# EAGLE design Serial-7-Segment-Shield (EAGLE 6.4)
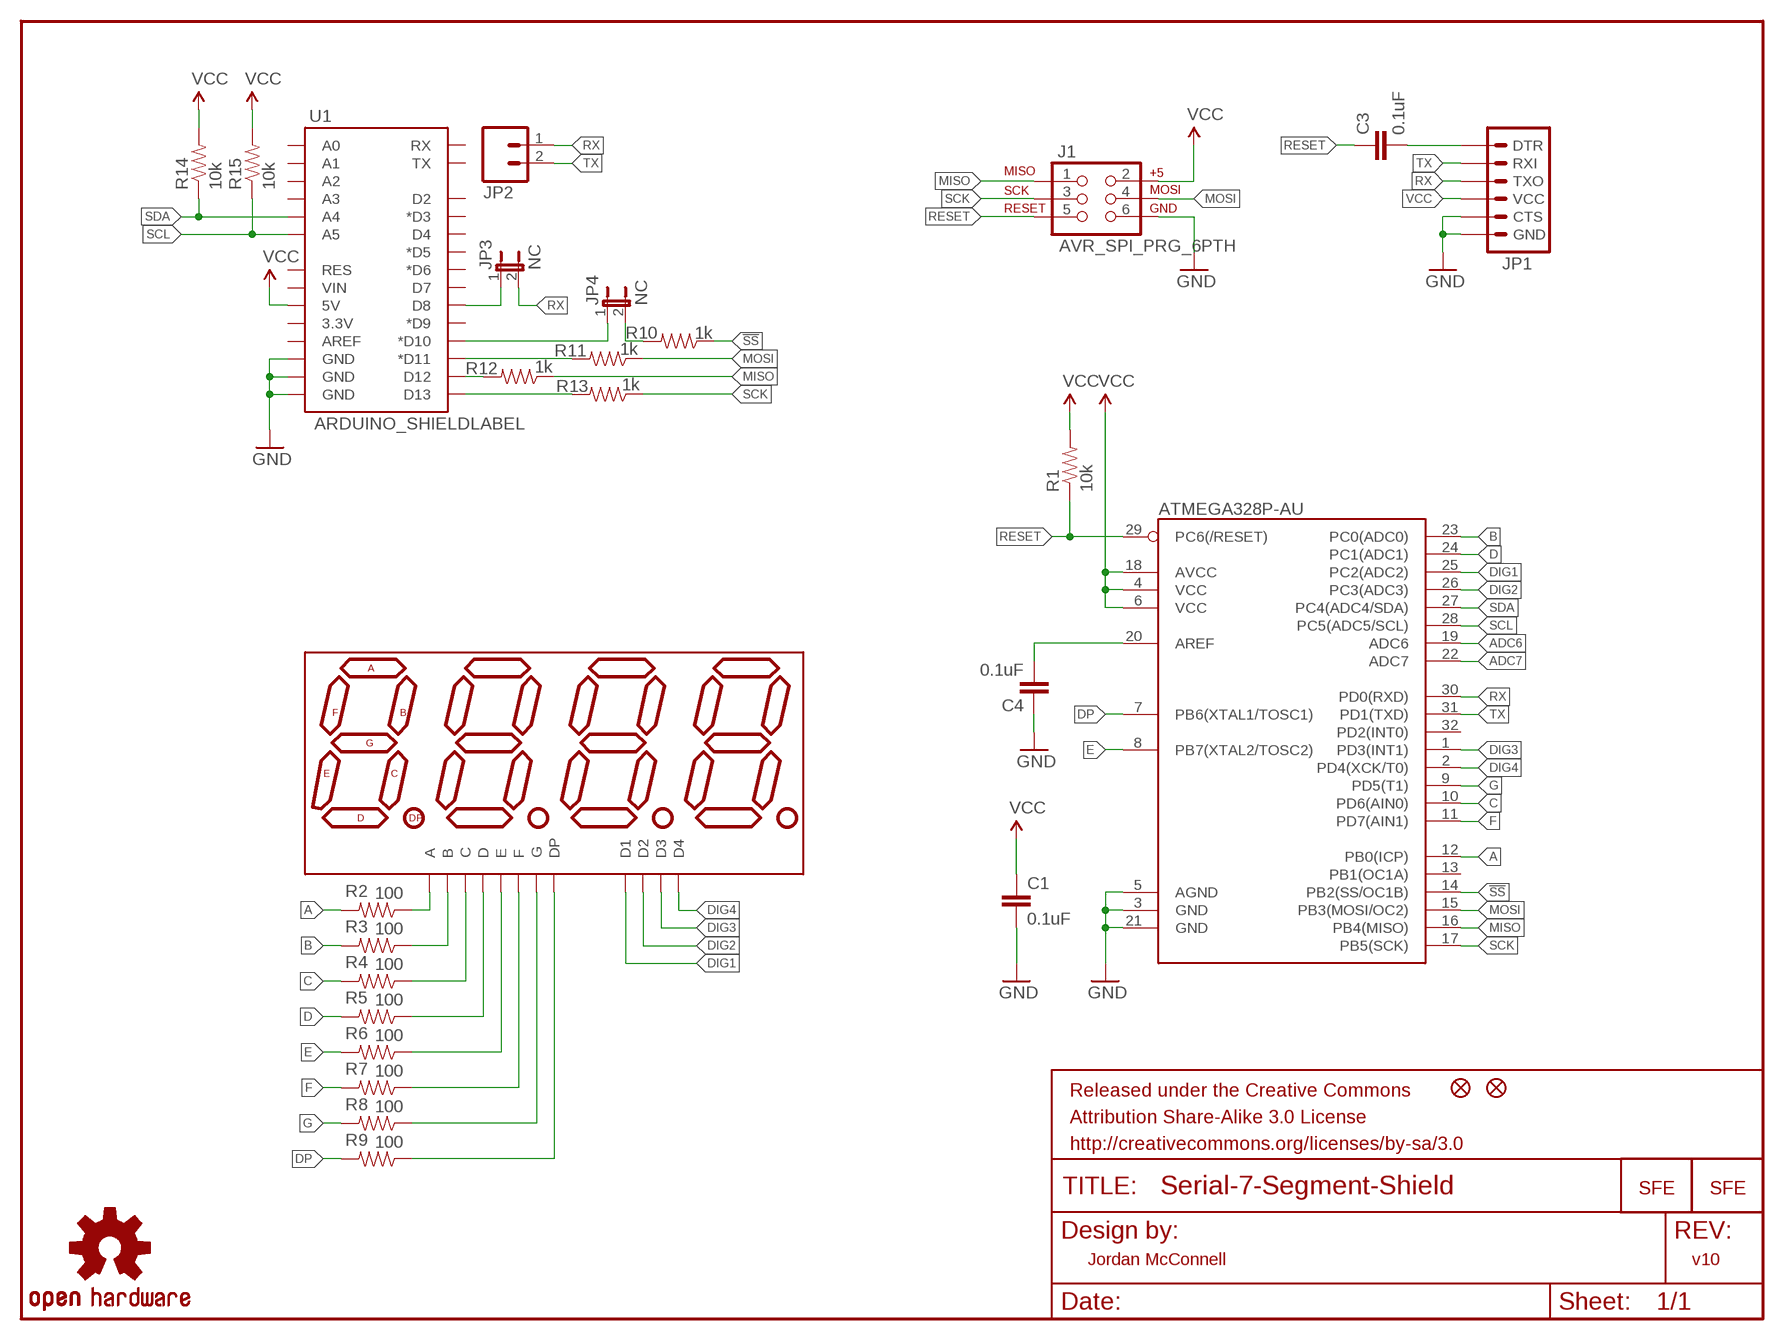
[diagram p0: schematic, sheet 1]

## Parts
ATMEGA328P-AU  ATMEGA328P-AU  ATMEGA168  [TQFP32-08]
C1  0.1uF  CAP0402-CAP  [0402-CAP]
C3  0.1uF  CAP0402-CAP  [0402-CAP]
C4  0.1uF  CAP0402-CAP  [0402-CAP]
FRAME1  FRAME-LETTER  [CREATIVE_COMMONS]
J1  AVR_SPI_PRG_6PTH  [2X3]
JP1  ARDUINO_SERIAL_PROGRAMPTH  [1X06]
JP2  M02PTH  [1X02]
JP3  NC  JUMPER-2SMD-NC  [SJ_2S]
JP4  NC  JUMPER-2SMD-NC  [SJ_2S]
JP9  FIDUCIALUFIDUCIAL  [MICRO-FIDUCIAL]
JP10  FIDUCIALUFIDUCIAL  [MICRO-FIDUCIAL]
LOGO1  LOGO-SFENEW  [SFE-NEW-WEBLOGO]
LOGO2  LOGO-SFENEW  [SFE-NEW-WEBLOGO]
R1  10k  RESISTOR0402-RES  [0402-RES]
R2  100  RESISTOR0402-RES  [0402-RES]
R3  100  RESISTOR0402-RES  [0402-RES]
R4  100  RESISTOR0402-RES  [0402-RES]
R5  100  RESISTOR0402-RES  [0402-RES]
R6  100  RESISTOR0402-RES  [0402-RES]
R7  100  RESISTOR0402-RES  [0402-RES]
R8  100  RESISTOR0402-RES  [0402-RES]
R9  100  RESISTOR0402-RES  [0402-RES]
R10  1k  RESISTOR0402-RES  [0402-RES]
R11  1k  RESISTOR0402-RES  [0402-RES]
R12  1k  RESISTOR0402-RES  [0402-RES]
R13  1k  RESISTOR0402-RES  [0402-RES]
R14  10k  RESISTOR0402-RES  [0402-RES]
R15  10k  RESISTOR0402-RES  [0402-RES]
U1  ARDUINO_SHIELDLABEL  [DUEMILANOVE_SHIELD]
U$1  7-SEGMENT-4DIGIT-COUNTERPTH  [7-SEGMENT-4DIGIT-COUNTER]
U$4  OSHW-LOGOS  [OSHW-LOGO-S]

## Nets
!SS: ATMEGA328P-AU.14(PB2(SS/OC1B)) R10.1
A: ATMEGA328P-AU.12(PB0(ICP)) R2.2
ADC6: ATMEGA328P-AU.19(ADC6)
ADC7: ATMEGA328P-AU.22(ADC7)
B: ATMEGA328P-AU.23(PC0(ADC0)) R3.2
C: ATMEGA328P-AU.10(PD6(AIN0)) R4.2
D: ATMEGA328P-AU.24(PC1(ADC1)) R5.2
DIG1: ATMEGA328P-AU.25(PC2(ADC2)) U$1.12(D1)
DIG2: ATMEGA328P-AU.26(PC3(ADC3)) U$1.9(D2)
DIG3: ATMEGA328P-AU.1(PD3(INT1)) U$1.8(D3)
DIG4: ATMEGA328P-AU.2(PD4(XCK/T0)) U$1.6(D4)
DP: ATMEGA328P-AU.7(PB6(XTAL1/TOSC1)) R9.2
E: ATMEGA328P-AU.8(PB7(XTAL2/TOSC2)) R6.2
F: ATMEGA328P-AU.11(PD7(AIN1)) R7.2
G: ATMEGA328P-AU.9(PD5(T1)) R8.2
GND: ATMEGA328P-AU.3(GND) ATMEGA328P-AU.5(AGND) ATMEGA328P-AU.21(GND) C1.2 C4.1 J1.6 JP1.5(CTS) JP1.6(GND) U1.GND@0(GND) U1.GND@1(GND) U1.GND@2(GND)
MISO: ATMEGA328P-AU.16(PB4(MISO)) J1.1 R12.1
MOSI: ATMEGA328P-AU.15(PB3(MOSI/OC2)) J1.4 R11.1
N$1: ATMEGA328P-AU.20(AREF) C4.2
N$2: R13.2 U1.D13
N$3: R12.2 U1.D12
N$4: R11.2 U1.D11(*D11)
N$5: JP4.2 R10.2
N$6: JP4.1 U1.D10(*D10)
N$7: JP3.1 U1.D8
N$11: R2.1 U$1.11(A)
N$12: R3.1 U$1.7(B)
N$13: C3.2 JP1.1(DTR)
N$14: R4.1 U$1.4(C)
N$15: R5.1 U$1.2(D)
N$16: R6.1 U$1.1(E)
N$17: R7.1 U$1.10(F)
N$18: R8.1 U$1.5(G)
N$19: R9.1 U$1.3(DP)
RESET: ATMEGA328P-AU.29(PC6(/RESET)) C3.1 J1.5 R1.1
RX: ATMEGA328P-AU.30(PD0(RXD)) JP1.3(TXO) JP2.1 JP3.2
SCK: ATMEGA328P-AU.17(PB5(SCK)) J1.3 R13.1
SCL: ATMEGA328P-AU.28(PC5(ADC5/SCL)) R15.1 U1.A5
SDA: ATMEGA328P-AU.27(PC4(ADC4/SDA)) R14.1 U1.A4
TX: ATMEGA328P-AU.31(PD1(TXD)) JP1.2(RXI) JP2.2
VCC: ATMEGA328P-AU.4(VCC) ATMEGA328P-AU.6(VCC) ATMEGA328P-AU.18(AVCC) C1.1 J1.2 JP1.4(VCC) R1.2 R14.2 R15.2 U1.5V
Unconnected: ATMEGA328P-AU.13(PB1(OC1A)) ATMEGA328P-AU.32(PD2(INT0)) U1.3.3V U1.A0 U1.A1 U1.A2 U1.A3 U1.AREF U1.D2 U1.D3(*D3) U1.D4 U1.D5(*D5) U1.D6(*D6) U1.D7 U1.D9(*D9) U1.RES U1.RX U1.TX U1.VIN

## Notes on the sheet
- Jordan McConnell | v10

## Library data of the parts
ATMEGA328P-AU = SparkFun:ATMEGA168
C1 = SparkFun:CAP: Capacitor
C3 C4 = SparkFun-Passives:CAP: Capacitor
FRAME1 = SparkFun-Aesthetics:FRAME-LETTER: Schematic Frame
J1 = SparkFun-Connectors:AVR_SPI_PRG_6: AVR ISP 6 Pin This is the reduced ISP connector for AVR programming. Common on Arduino. This footprint will take up less PCB space and can be used with a 10-pin to 6-pin adapter such as SKU: BOB-08508
JP1 = SparkFun-Connectors:ARDUINO_SERIAL_PROGRAM: FTDI connector footprints
JP2 = SparkFun-Connectors:M02: Header 2
JP3 JP4 = SparkFun-Passives:JUMPER-2: Jumper
JP9 JP10 = SparkFun:FIDUCIAL: Fiducial Alignment Points
LOGO1 LOGO2 = SparkFun-Aesthetics:LOGO-SFE: Spark Fun Electronics PCB Logo
R1-R15 = SparkFun:RESISTOR: Resistor
U1 = SparkFun-Boards:ARDUINO_SHIELD: Arduino shield footprint
U$1 = SparkFun-Displays:7-SEGMENT-4DIGIT-COUNTER
U$4 = SparkFun-Aesthetics:OSHW-LOGO: Open Source Hardware Logo This logo indicates the piece of hardware it is found on incorporates a OSHW license and/or adheres to the definition of open source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

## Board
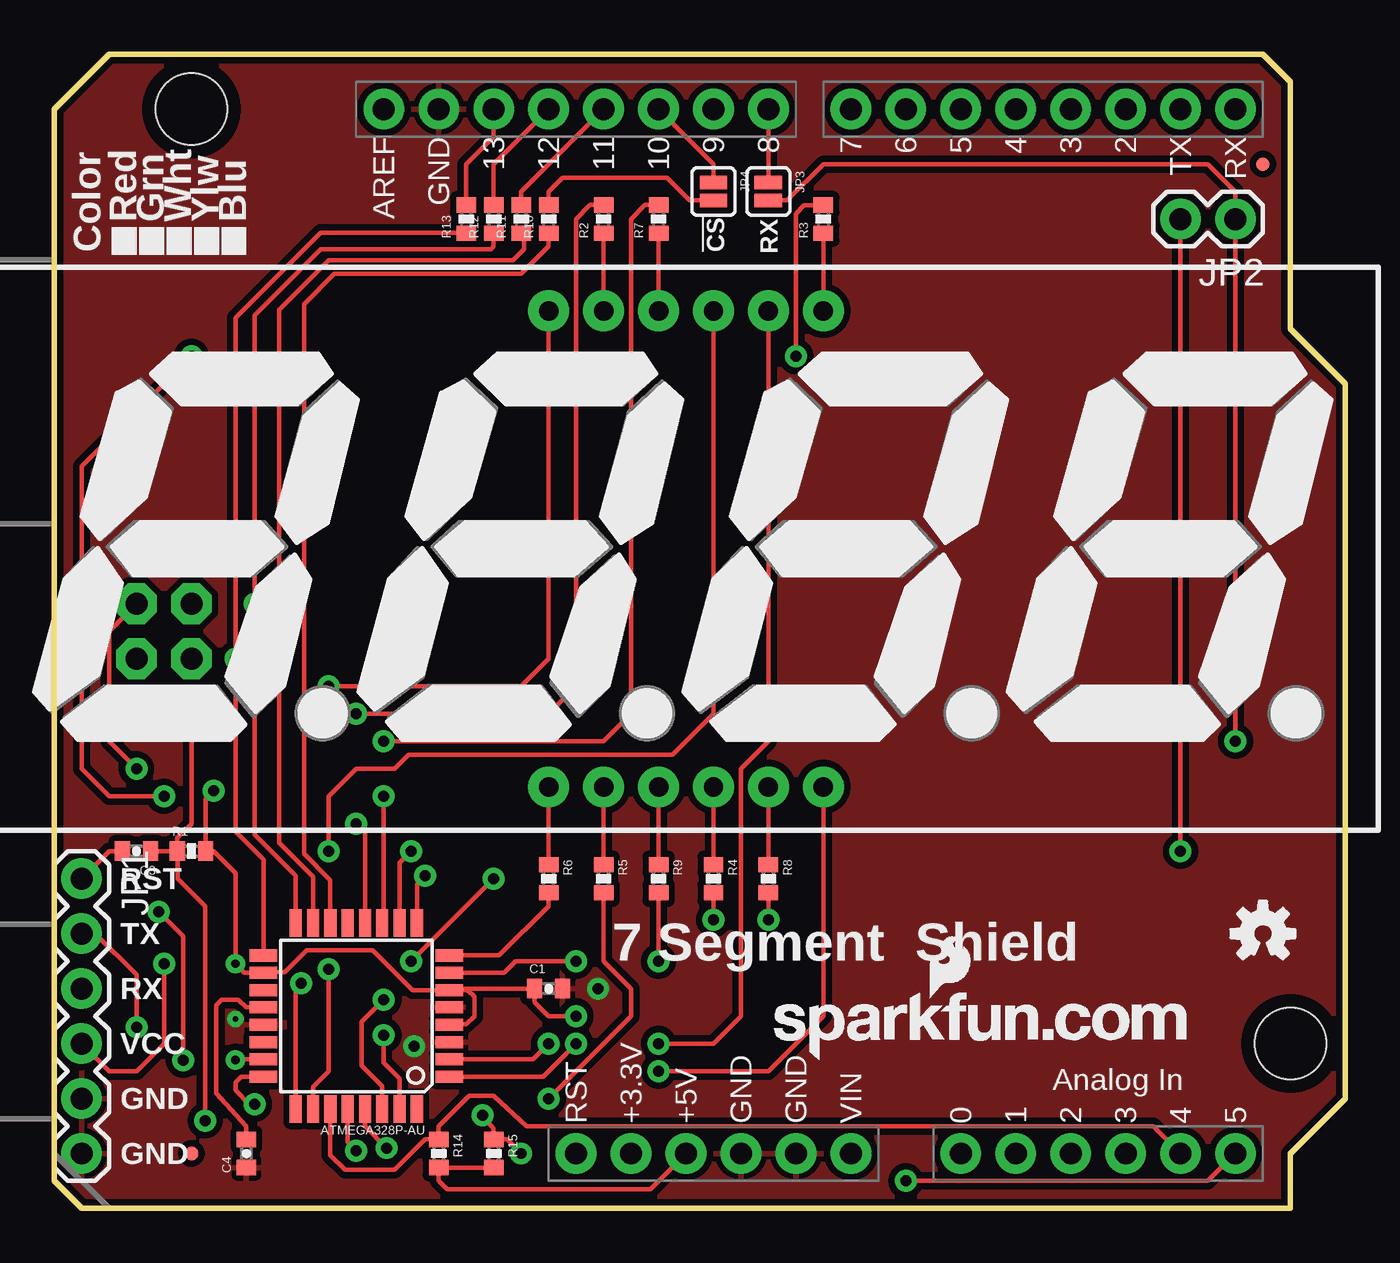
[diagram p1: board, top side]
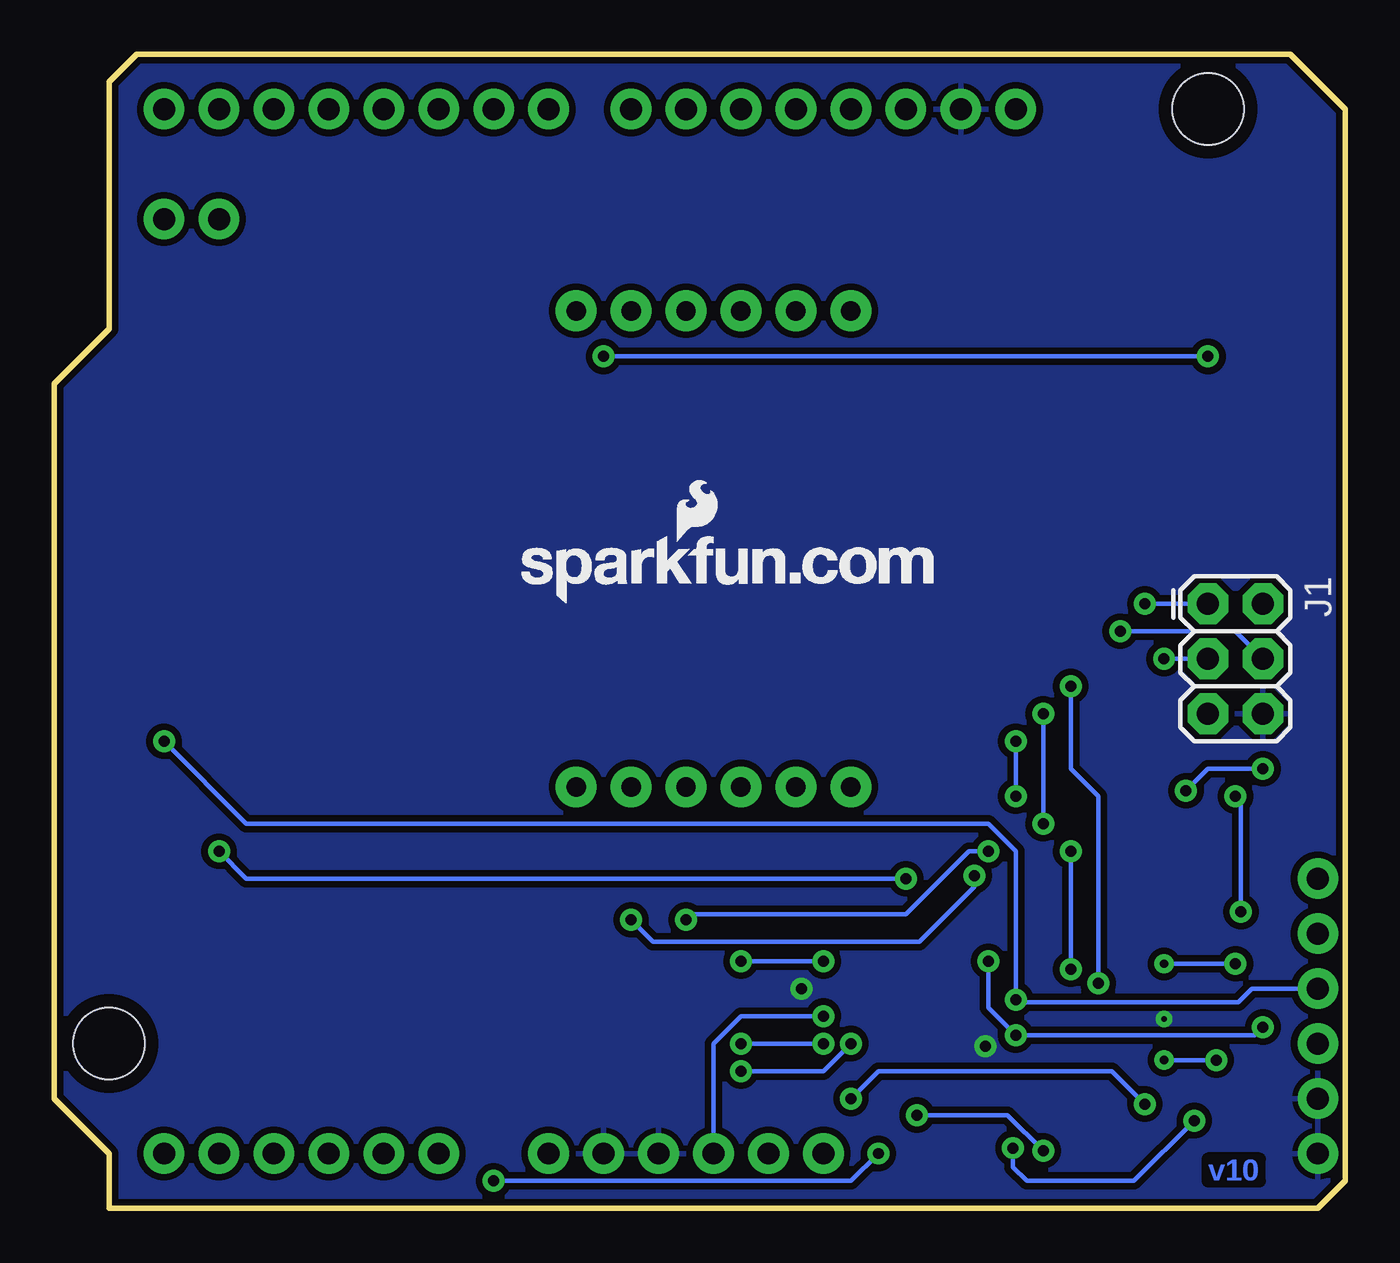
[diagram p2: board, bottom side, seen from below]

Size 59.69 x 53.34 mm. Coordinates in mm from the lower left corner, seen from the top.
Outline: 0,1.27 0,50.8 2.54,53.34 55.88,53.34 57.15,52.07 57.15,40.64 59.69,38.1 59.69,5.08 57.15,2.54 57.15,0 1.27,0 0,1.27
Copper layers (1*16): Top 0.035mm / dielectric 1.5mm / Bottom 0.035mm
Design rules "default": minimum track width 8mil, minimum drill 20mil, track to track 8mil, track to pad 8mil, pad to pad 8mil, via to via 8mil, smd to smd 8mil, copper to edge 8mil, drill to drill 8mil, minimum pad ring 12mil, minimum via ring 10mil, stop-mask expansion 4mil, vias tented up to drill 20mil, thermal gap 10mil

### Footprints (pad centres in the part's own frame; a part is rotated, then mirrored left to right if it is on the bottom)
TQFP32-08 = smd 1.27 x 0.559: 1 -4.293,2.8; 2 -4.293,2; 3 -4.293,1.2; 4 -4.293,0.4; 5 -4.293,-0.4; 6 -4.293,-1.2; 7 -4.293,-2; 8 -4.293,-2.8; 17 4.293,-2.8; 18 4.293,-2; 19 4.293,-1.2; 20 4.293,-0.4; 21 4.293,0.4; 22 4.293,1.2; 23 4.293,2; 24 4.293,2.8 | smd 0.559 x 1.27: 9 -2.8,-4.293; 10 -2,-4.293; 11 -1.2,-4.293; 12 -0.4,-4.293; 13 0.4,-4.293; 14 1.2,-4.293; 15 2,-4.293; 16 2.8,-4.293; 25 2.8,4.293; 26 2,4.293; 27 1.2,4.293; 28 0.4,4.293; 29 -0.4,4.293; 30 -1.2,4.293; 31 -2,4.293; 32 -2.8,4.293
0402-CAP = smd 0.7 x 0.9: 1 -0.65,0; 2 0.65,0
2X3 = drill 1.016 pad 1.88 octagon: 1 0,0; 2 0,2.54; 3 2.54,0; 4 2.54,2.54; 5 5.08,0; 6 5.08,2.54
1X06 = drill 1.016 pad 1.88: 1 0,0; 2 2.54,0; 3 5.08,0; 4 7.62,0; 5 10.16,0; 6 12.7,0
1X02 = drill 1.016 pad 1.88: 1 0,0; 2 2.54,0
SJ_2S = smd 0.635 x 1.27: 1 -0.412,0; 2 0.412,0
MICRO-FIDUCIAL = smd 0.635 x 0.635: 1 0,0
0402-RES = smd 0.7 x 0.9: 1 -0.65,0; 2 0.65,0
DUEMILANOVE_SHIELD = drill 1.016 pad 1.88: 3.3V 50.8,26.67; 5V 50.8,29.21; A0 50.8,41.91; A1 50.8,44.45; A2 50.8,46.99; A3 50.8,49.53; A4 50.8,52.07; A5 50.8,54.61; AREF 2.54,15.24; D2 2.54,49.53; D3 2.54,46.99; D4 2.54,44.45; D5 2.54,41.91; D6 2.54,39.37; D7 2.54,36.83; D8 2.54,33.02; D9 2.54,30.48; D10 2.54,27.94; D11 2.54,25.4; D12 2.54,22.86; D13 2.54,20.32; GND@0 50.8,31.75; GND@1 50.8,34.29; GND@2 2.54,17.78; RES 50.8,24.13; RX 2.54,54.61; TX 2.54,52.07; VIN 50.8,36.83 | hole 3.302: 45.72,57.15; 2.54,6.35
7-SEGMENT-4DIGIT-COUNTER = drill 0.9 pad 1.88: 1 -6.35,-10.998; 2 -3.81,-10.998; 3 -1.27,-10.998; 4 1.27,-10.998; 5 3.81,-10.998; 6 6.35,-10.998; 7 6.35,10.998; 8 3.81,10.998; 9 1.27,10.998; 10 -1.27,10.998; 11 -3.81,10.998; 12 -6.35,10.998

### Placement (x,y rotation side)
ATMEGA328P-AU  13.97,8.89 180 top
C1  22.86,10.16 0 top
C3  3.81,16.51 180 top
C4  8.89,2.54 90 top
FRAME1  not placed on the board
J1  6.35,27.94 270 bottom
JP1  1.27,15.24 270 top
JP2  54.61,45.72 180 top
JP3  33.02,46.99 270 top
JP4  30.48,46.99 270 top
JP9  55.88,48.26 0 top
JP10  6.35,2.54 0 top
LOGO1  33.27,6.86 0 top
LOGO2  38.1,27.94 0 bottom
R1  6.35,16.51 0 top
R2  25.4,45.72 90 top
R3  35.56,45.72 90 top
R4  30.48,15.24 270 top
R5  25.4,15.24 270 top
R6  22.86,15.24 270 top
R7  27.94,45.72 90 top
R8  33.02,15.24 270 top
R9  27.94,15.24 270 top
R10  22.86,45.72 90 top
R11  21.59,45.72 90 top
R12  20.32,45.72 90 top
R13  19.05,45.72 90 top
R14  17.78,2.54 270 top
R15  20.32,2.54 270 top
U1  0,53.34 270 top
U$1  29.21,30.48 0 top
U$4  55.88,12.7 0 top

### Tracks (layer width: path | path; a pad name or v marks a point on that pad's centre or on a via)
!SS
  Top 0.203: ATMEGA328P-AU.14 12.77,15.17 11.56,16.38 11.56,41.78 12.95,43.18 21.59,43.18 22.86,44.45 R10.1
A  (via drill 0.51)
  Top 0.203: R2.2 24.78,46.37 24.13,45.72 24.13,24.13 22.86,22.86 v13.97,22.86 | v13.97,17.78 14.37,17.38 ATMEGA328P-AU.12
  Bottom 0.203: v13.97,22.86 v13.97,17.78
B  (via drill 0.38, 0.51)
  Top 0.203: ATMEGA328P-AU.23 8.41,6.89 v8.38,6.86 | v5.97,6.86 5.97,12.57 v4.83,13.72 | v6.35,39.37 5.08,38.1 1.27,34.29 1.27,20.32 2.54,19.05 v5.08,19.05 | v34.29,39.37 34.29,45.97 34.67,46.35 35.55,46.35 R3.2
  Bottom 0.203: v8.38,6.86 v5.97,6.86 | v4.83,13.72 4.83,18.8 v5.08,19.05 | v6.35,39.37 v34.29,39.37
C  (via drill 0.51)
  Top 0.203: R4.2 v30.48,13.34 | v16.51,16.51 15.97,15.97 ATMEGA328P-AU.10
  Bottom 0.203: v30.48,13.34 30.23,13.59 20.32,13.59 17.4,16.51 v16.51,16.51
D  (via drill 0.51)
  Top 0.203: v22.86,5.08 26.67,8.89 26.67,10.16 25.4,11.43 R5.2 | v9.27,4.83 9.02,4.83 8.38,5.46 8.38,5.84 8.64,6.1 ATMEGA328P-AU.24
  Bottom 0.203: v22.86,5.08 21.59,6.35 10.79,6.35 v9.27,4.83
DIG1  (via drill 0.51)
  Top 0.203: U$1.12 22.86,25.4 21.59,24.13 v12.7,24.13 | ATMEGA328P-AU.25 11.17,10.15 v11.43,10.41
  Bottom 0.203: v11.43,10.41 11.43,19.05 12.7,20.32 v12.7,24.13
DIG2  (via drill 0.51)
  Top 0.203: U$1.9 30.48,22.86 28.57,20.95 16.38,20.95 15.75,20.32 13.97,20.32 12.7,19.05 v12.7,16.51 | v12.7,11.05 12.7,6.35 11.97,5.62 ATMEGA328P-AU.26
  Bottom 0.203: v12.7,16.51 v12.7,11.05
DIG3  (via drill 0.51)
  Top 0.203: U$1.8 33.02,21.59 31.75,20.32 31.75,8.89 30.48,7.62 v27.94,7.62 | v24.13,7.62 22.6,6.09 ATMEGA328P-AU.1
  Bottom 0.203: v27.94,7.62 v24.13,7.62
DIG4  (via drill 0.51)
  Top 0.203: U$1.6 35.56,8.89 33.02,6.35 v27.94,6.35 | v22.86,7.62 22.13,6.89 ATMEGA328P-AU.2
  Bottom 0.203: v22.86,7.62 24.13,6.35 v27.94,6.35
DP  (via drill 0.51)
  Top 0.203: R9.2 v27.94,11.43 | v24.13,11.43 21.34,11.43 20.8,10.89 ATMEGA328P-AU.7
  Bottom 0.203: v27.94,11.43 v24.13,11.43
E
  Top 0.203: R6.2 22.86,13.97 20.58,11.69 ATMEGA328P-AU.8
F  (via drill 0.51)
  Top 0.203: R7.2 27.32,46.37 26.67,45.72 26.67,22.86 25.4,21.59 v15.24,21.59 | v15.24,19.05 15.24,13.25 ATMEGA328P-AU.11
  Bottom 0.203: v15.24,21.59 v15.24,19.05
G  (via drill 0.51)
  Top 0.203: v17.14,15.37 16.77,14.99 ATMEGA328P-AU.9 | R8.2 v33.02,13.34
  Bottom 0.203: v17.14,15.37 17.14,14.86 19.68,12.32 32,12.32 v33.02,13.34
GND  (via drill 0.25, 0.51)
  other vias: 25.15,10.16 16.64,7.49 8.38,8.76
  pour Top (isolate 0.305): 0,1.27 0,50.8 2.54,53.34 55.88,53.34 57.15,52.07 57.15,40.64 59.69,38.1 59.69,5.08 57.15,2.54 57.15,0 1.27,0
  pour Bottom (isolate 0.305): 0,1.27 0,50.8 2.54,53.34 55.88,53.34 57.15,52.07 57.15,40.64 59.69,38.1 59.69,5.08 57.15,2.54 57.15,0 1.27,0
MISO  (via drill 0.51)
  Top 0.203: ATMEGA328P-AU.16 11.17,15.37 9.27,17.27 v9.27,27.94 9.27,41.27 12.32,44.32 20.19,44.32 20.32,44.45 R12.1
  Bottom 0.203: J1.1 v9.27,27.94
MOSI  (via drill 0.51)
  Top 0.203: ATMEGA328P-AU.15 11.97,15.34 10.41,16.89 v10.41,26.67 10.41,41.53 12.7,43.81 13.84,43.81 21.21,43.81 21.72,44.32 21.72,44.94 R11.1
  Bottom 0.203: J1.4 5.08,26.67 v10.41,26.67
N$1
  Top 0.203: C4.2 8.89,3.81 7.49,5.33 7.49,9.4 7.75,9.65 8.51,9.65 8.87,9.29 ATMEGA328P-AU.20
N$2
  Top 0.203: R13.2 19.05,48.26 20.32,49.53 U1.D13
N$3
  Top 0.203: R12.2 20.32,48.26 U1.D12
N$4
  Top 0.203: R11.2 21.59,46.99 U1.D11
N$5
  Top 0.203: JP4.2 29.37,46.58 28.32,47.62 23.5,47.62 22.86,46.99 R10.2
N$6
  Top 0.203: JP4.1 30.48,48.26 U1.D10
N$7
  Top 0.203: JP3.1 U1.D8
N$11
  Top 0.203: U$1.11 R2.1
N$12
  Top 0.203: U$1.7 R3.1
N$13
  Top 0.203: C3.2 2.54,16.51 JP1.1
N$14
  Top 0.203: U$1.4 R4.1
N$15
  Top 0.203: R5.1 U$1.2
N$16
  Top 0.203: R6.1 U$1.1
N$17
  Top 0.203: U$1.10 R7.1
N$18
  Top 0.203: R8.1 U$1.5
N$19
  Top 0.203: R9.1 U$1.3
RESET  (via drill 0.51)
  Top 0.203: ATMEGA328P-AU.29 14.37,3.79 v15.37,2.79 | v6.99,4.06 6.99,13.97 5.71,15.24 5.71,16.5 R1.1 | R1.1 C3.1 | R1.1 5.7,17.13 6.35,17.78 J1.5
  Bottom 0.203: v15.37,2.79 15.37,1.91 14.73,1.27 9.78,1.27 v6.99,4.06
RX  (via drill 0.51)
  Top 0.203: ATMEGA328P-AU.30 15.17,5.66 14.22,6.6 14.22,8.64 v15.24,9.65 | v54.61,21.59 JP2.1 54.61,46.99 53.34,48.26 35.56,48.26 33.88,46.58 JP3.2
  Bottom 0.203: v54.61,21.59 50.8,17.78 16.51,17.78 15.24,16.51 v15.24,9.65 15.11,9.53 4.95,9.53 4.32,10.16 JP1.3
SCK  (via drill 0.51)
  Top 0.203: ATMEGA328P-AU.17 9.68,16.1 8.38,17.4 v8.38,25.4 8.38,41.15 12.32,45.09 19.04,45.09 R13.1
  Bottom 0.203: J1.3 v8.38,25.4
SCL  (via drill 0.51)
  Top 0.203: U1.A5 53.34,1.27 v39.37,1.27 | v19.81,4.32 20.32,3.68 R15.1 20.94,3.19 v21.59,2.54 | v13.97,2.67 13.57,3.07 ATMEGA328P-AU.28
  Bottom 0.203: v19.81,4.32 15.62,4.32 v13.97,2.67 | v21.59,2.54 22.86,1.27 v39.37,1.27
SDA
  Top 0.203: U1.A4 50.8,3.81 21.84,3.81 20.32,5.21 19.18,5.21 17.78,3.81 R14.1 17.16,3.19 15.75,1.78 13.46,1.78 12.77,2.47 ATMEGA328P-AU.27
TX  (via drill 0.51)
  Top 0.203: v16.51,11.43 v20.32,15.24 | ATMEGA328P-AU.31 15.97,6 15.24,6.73 v15.24,8 | JP1.2 1.91,12.7 3.81,10.79 v3.81,8.38 | v52.07,16.51 JP2.2
  Bottom 0.203: v20.32,15.24 50.8,15.24 v52.07,16.51 | v16.51,11.43 16.51,9.27 v15.24,8 4.19,8 v3.81,8.38
VCC  (via drill 0.38, 0.51)
  Top 0.203: ATMEGA328P-AU.6 18.33,10.16 C1.1 22.21,9.54 22.86,8.89 v24.13,8.89 | ATMEGA328P-AU.6 16.58,10.09 14.73,11.94 11.68,11.94 10.67,10.92 9.71,10.92 ATMEGA328P-AU.18 8.79,10.89 v8.38,11.3 8.38,15.49 7.37,16.51 R1.2 7,18.94 v7.37,19.3 | R15.2 R14.2 17.78,1.27 18.16,0.89 27.56,0.89 U1.5V | ATMEGA328P-AU.6 19.12,10.09 19.43,9.78 19.43,8.89 19.05,8.51 18.28,8.51 ATMEGA328P-AU.4 | v5.08,11.3 5.08,7.62 3.81,6.35 2.54,6.35 JP1.4 | J1.2 2.54,26.67 2.54,21.59 v3.81,20.32
  Bottom 0.203: v24.13,8.89 27.94,8.89 29.21,7.62 U1.5V | v8.38,11.3 v5.08,11.3 | v3.81,20.32 6.35,20.32 v7.37,19.3

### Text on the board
Bottom: v10
tPlace: Red | Grn | Wht | Ylw | Blu | RX | Color | !CS | RST | TX | 7 Segment Shield | RX | VCC | GND | GND
tValues: Jordan McConnell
